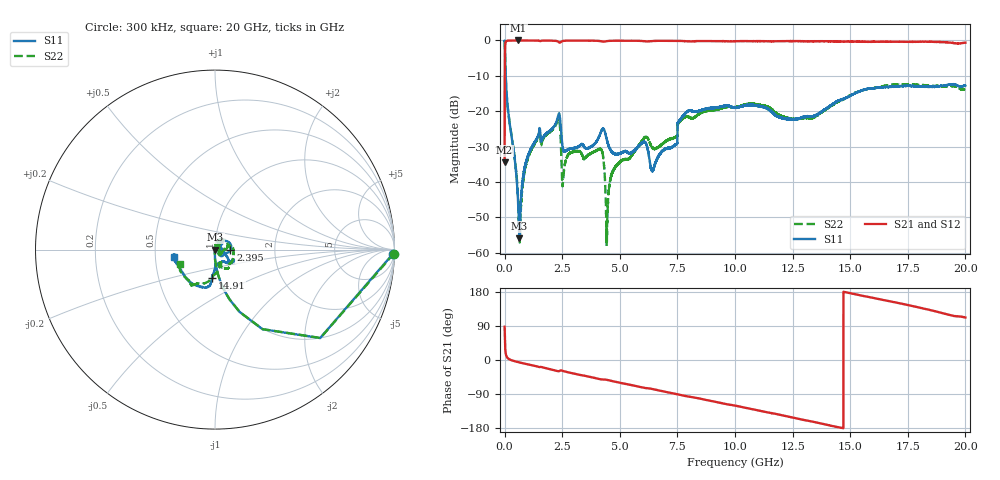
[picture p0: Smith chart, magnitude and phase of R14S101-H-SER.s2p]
!{R14S101}
!Johanson Technology Inc.
!www.johansontechnology.com
!Test Board Conditions:
!Substrate Type  RO4350B
!Substrate Thickness  20 mil
!Substrate Dk  3.66
!TL Type: GCPW
!TL Trace Width  36 mil
!TL Gap  12 mil
!Electrode orientation  Horizontal
!DUT TOPOLOGY	SERIES
!Mounting Pad LxW  26x36 mil
! Created Wed Nov 25 17:33:21 2020
! 2 Port Network Data from SP1.SP block
! freq  magS11  angS11  magS21  angS21  magS12  angS12  magS22  angS22
# khz S ma R 50
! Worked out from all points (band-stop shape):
!   20001 points, 300 kHz to 20 GHz, reference 50 ohm
!   highest |S21| = 0.00 dB at 594.3 MHz (marker M1); lowest = -34.5 dB at 300 kHz (marker M2)
!   |S21| within 3 dB of the highest: 15.99 MHz to end of sweep
!   lowest |S11| = -55.9 dB at 643.3 MHz (marker M3), VSWR 1.00, Z = 50.2 + j0.00145 ohm
!   |S11| at or under -10 dB: 47.33 MHz to end of sweep
!   |S22| runs from -58.1 to 0.0 dB; largest |S21 - S12| = 0.018
!   S11 on the Smith chart (normalised r, x): 300 kHz: 26, -81; 2.395 GHz: 1.19, -0.01; 14.91 GHz: 0.92, -0.30; 20 GHz: 0.63, -0.06
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300  0.9927 -1.3  0.01886 87.7  0.01892 88.5  0.9969 -1.3
109300  0.1411 -82.9  0.9897 6.9  0.989 6.9  0.1418 -83.0
594300  0.004515 -76.1  0.9999 -5.7  0.9987 -5.7  0.005326 -113.2
643300  0.001594 0.5  0.9984 -6.5  0.9999 -6.4  0.001777 -170.2
928300  0.01889 68.8  0.9982 -10.4  0.9983 -10.5  0.01765 89.8
1437300  0.04366 60.2  0.9955 -17.4  0.9955 -17.4  0.04168 79.1
2395300  0.08594 -2.4  0.9314 -28.5  0.9317 -28.5  0.06568 5.4
2562300  0.02747 0.0  0.9863 -29.4  0.9872 -29.3  0.01279 71.5
3334300  0.0341 1.2  0.9904 -40.0  0.9909 -40.1  0.02531 77.6
4186300  0.05144 -16.0  0.9752 -51.1  0.9753 -51.1  0.029 36.4
4463300  0.03651 -52.6  0.9796 -52.7  0.9796 -52.7  0.003465 140.7
4884300  0.02475 -24.5  0.993 -58.5  0.9929 -58.4  0.01716 71.3
6095300  0.03644 -1.7  0.9746 -73.8  0.9749 -73.8  0.04294 -21.8
6398300  0.01468 14.9  0.9786 -76.4  0.9806 -76.3  0.03093 -49.1
6667300  0.0226 49.0  0.988 -79.9  0.9875 -79.9  0.03128 -44.9
7399300  0.03352 48.6  0.988 -89.2  0.9879 -89.2  0.04254 -58.1
7936300  0.09934 -40.8  0.973 -96.0  0.9728 -95.9  0.0832 11.0
1.00003e7  0.1122 -31.7  0.9731 -120.3  0.9737 -120.4  0.1138 -44.8
1.33343e7  0.08365 -88.0  0.9734 -162.4  0.9749 -162.3  0.07932 -73.8
1.49053e7  0.1589 -95.8  0.9658 177.6  0.9652 177.4  0.1605 -96.7
1.66673e7  0.2191 -108.8  0.9622 155.6  0.9555 155.4  0.2341 -121.8
2e7  0.2311 -169.0  0.93 112.1  0.9294 112.3  0.2085 -158.3
